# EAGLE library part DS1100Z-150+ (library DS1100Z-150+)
Delay Lines / Timing Elements 5-Tap Economy Timing Element (Delay Line) Source: Datasheet
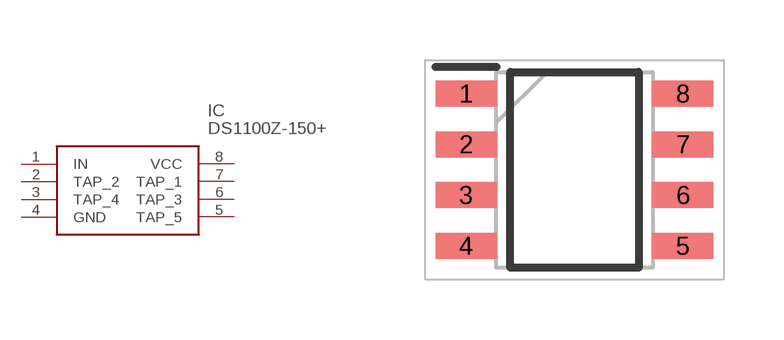
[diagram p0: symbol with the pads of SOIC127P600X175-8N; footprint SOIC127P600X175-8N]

Designator prefix IC

## DS1100Z-150+ (Description: Delay Lines / Timing Elements 5-Tap Economy Timing Element (Delay Line); Height: 1.75mm; Manufacturer_Name: Analog Devices; Manufacturer_Part_Number: DS1100Z-150+; Mouser_Part_Number: 700-DS1100Z-150; Mouser_Price-Stock: https://www.mouser.co.uk/ProductDetail/Maxim-Integrated/DS1100Z-150%2b?qs=Jw2w9zrI6w9cWpTP9DBTEQ%3D%3D)  [SOIC127P600X175-8N]
1  IN
2  TAP_2
3  TAP_4
4  GND
5  TAP_5
6  TAP_3
7  TAP_1
8  VCC

## Footprint SOIC127P600X175-8N (pad centres in mm)
S8+4
smd 1.525 x 0.65: 1 -2.712,1.905; 2 -2.712,0.635; 3 -2.712,-0.635; 4 -2.712,-1.905; 5 2.712,-1.905; 6 2.712,-0.635; 7 2.712,0.635; 8 2.712,1.905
